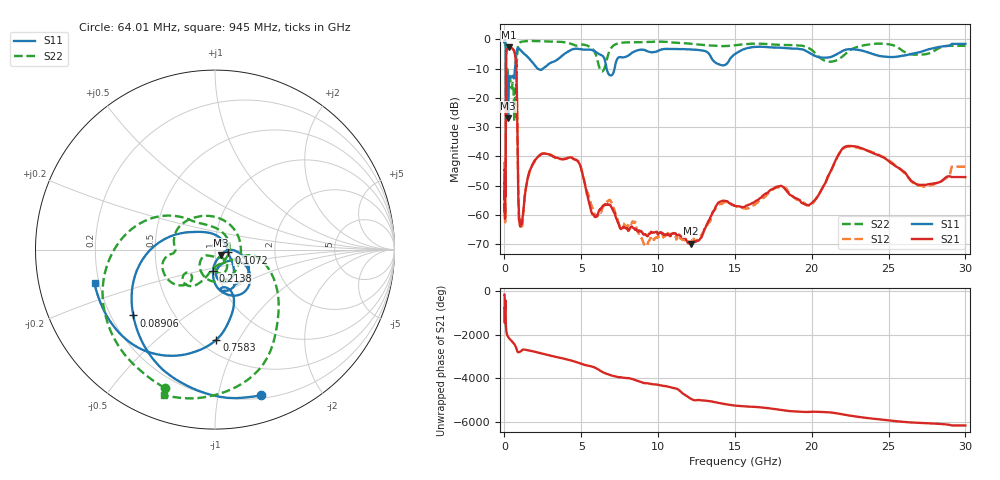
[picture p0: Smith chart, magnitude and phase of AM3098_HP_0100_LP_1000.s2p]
! Date/Time: Thu, Feb 28, 2019 8:35 AM
! Network Analyzer: Agilent Technologies E8364B Rev: A.07.50.67
! Sweep from 0.010 to 30.000 GHz, 1601 Points, Sweep Type: LOG
! Power Supply: 5.022 V, 0.002 A
# Hz S DB R 50
!freq MagS11 AngS11 MagS21 AngS21 MagS12 AngS12 MagS22 AngS22
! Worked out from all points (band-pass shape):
!   1601 points, 10 MHz to 30 GHz, reference 50 ohm
!   highest |S21| = -2.73 dB at 266.5 MHz (marker M1); lowest = -69.9 dB at 12.13 GHz (marker M2)
!   |S21| within 3 dB of the highest: 112.1 MHz to 705.9 MHz (593.8 MHz wide, 145 % of centre)
!   lowest |S11| = -26.9 dB at 237.5 MHz (marker M3), VSWR 1.09, Z = 53.4 - j3.22 ohm
!   |S11| at or under -10 dB: 95.98 MHz to 682.8 MHz (586.8 MHz wide, 151 % of centre); 2.159 GHz to 2.515 GHz (356 MHz wide, 15.2 % of centre); 6.648 GHz to 7.166 GHz (518.2 MHz wide, 7.5 % of centre)
!   |S22| runs from -28.0 to -0.5 dB; largest |S21 - S12| = 0.013
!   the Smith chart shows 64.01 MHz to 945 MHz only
!   S11 on the Smith chart (normalised r, x): 64.01 MHz: 0.23, -1.34; 89.06 MHz: 0.29, -0.33; 107.2 MHz: 1.16, -0.04; 213.8 MHz: 0.95, -0.23; 758.3 MHz: 0.61, -0.81; 945 MHz: 0.18, -0.13
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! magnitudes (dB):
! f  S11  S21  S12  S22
! 10 MHz  -0.4  -44.7  -42.6  -0.6
! 38.04 MHz  -0.5  -61.3  -59.3  -0.9
! 64.01 MHz  -1.4  -51.8  -52.9  -1.7
! 79.38 MHz  -2.4  -48.9  -48.7  -2.9
! 89.06 MHz  -4.7  -31.3  -31.1  -5.2
! 107.2 MHz  -22.4  -6.8  -6.9  -15.9
! 144.7 MHz  -17.1  -3.5  -3.5  -13.6
! 213.8 MHz  -18.6  -3.0  -2.9  -11.7
! 237.5 MHz  -26.9  -2.8  -2.8  -12.7
! 266.5 MHz  -18.3  -2.7  -2.7  -13.1
! 550.5 MHz  -12.7  -3.4  -3.4  -15.0
! 639.6 MHz  -12.7  -4.1  -4.0  -28.0
! 758.3 MHz  -6.0  -9.1  -9.0  -18.8
! 945 MHz  -3.1  -59.1  -61.9  -1.3
! 2.084 GHz  -9.6  -40.8  -40.5  -0.6
! 4.64 GHz  -3.2  -41.2  -41.0  -2.1
! 5.783 GHz  -3.7  -60.0  -58.3  -3.6
! 7.926 GHz  -5.9  -64.6  -63.8  -1.0
! 12.13 GHz  -3.4  -69.9  -69.8  -1.5
! 19.9 GHz  -4.8  -56.4  -56.9  -3.3
! 22.67 GHz  -3.4  -36.6  -36.8  -3.2
! 30 GHz  -1.5  -47.1  -43.5  -2.2
